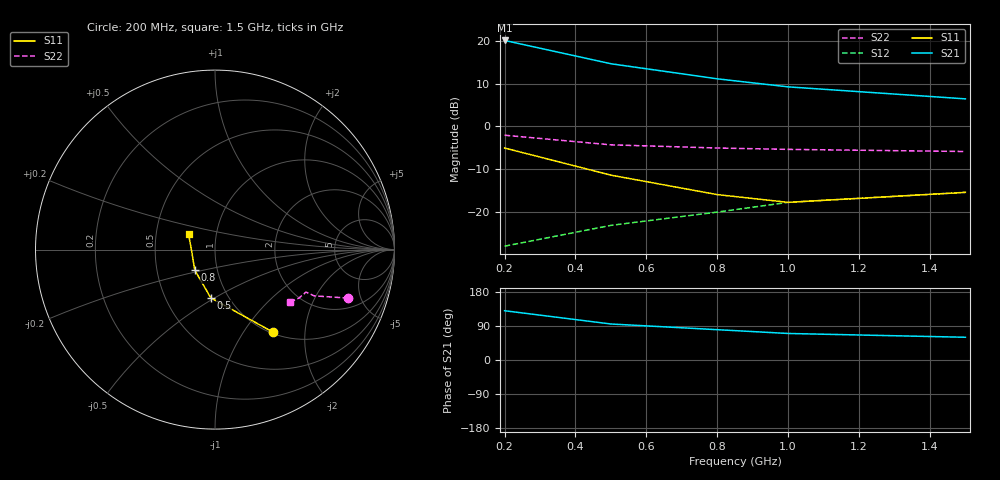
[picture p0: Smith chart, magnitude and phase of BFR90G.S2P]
!  BFR90G.S2P
!  BFR90
!  VCE=10V; IC=5mA
#  GHZ S MA R 50
!  S-PARAMETER DATA
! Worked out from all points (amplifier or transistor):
!   5 points, 200 MHz to 1.5 GHz, reference 50 ohm
!   highest |S21| = 20.1 dB at 200 MHz (marker M1)
!   |S21| within 3 dB of that: start of sweep to 365.5 MHz
!   unconditionally stable (mu >= 1): 665.3 MHz to end of sweep
!   at 200 MHz: K = 0.52, MSG = 24.0 dB, |S12| = -28.0 dB
!   at 800 MHz: K = 1.06, MAG = 14.1 dB, |S12| = -20.0 dB
!   at 1.5 GHz: K = 1.10, MAG = 9.0 dB, |S12| = -15.4 dB
!   S11 on the Smith chart (normalised r, x): 200 MHz: 1.02, -1.37; 500 MHz: 0.83, -0.48; 800 MHz: 0.78, -0.18; 1.5 GHz: 0.73, +0.13
0.2  0.56 -55.0  10.1 130.0  0.04 65.0  0.79 -20.0
0.5  0.27 -95.0  5.4 95.0  0.07 65.0  0.61 -25.0
0.8  0.16 -135.0  3.6 80.0  0.1 65.0  0.56 -25.0
1  0.13 -175.0  2.9 70.0  0.13 65.0  0.54 -30.0
1.5  0.17 150.0  2.1 60.0  0.17 70.0  0.51 -35.0
